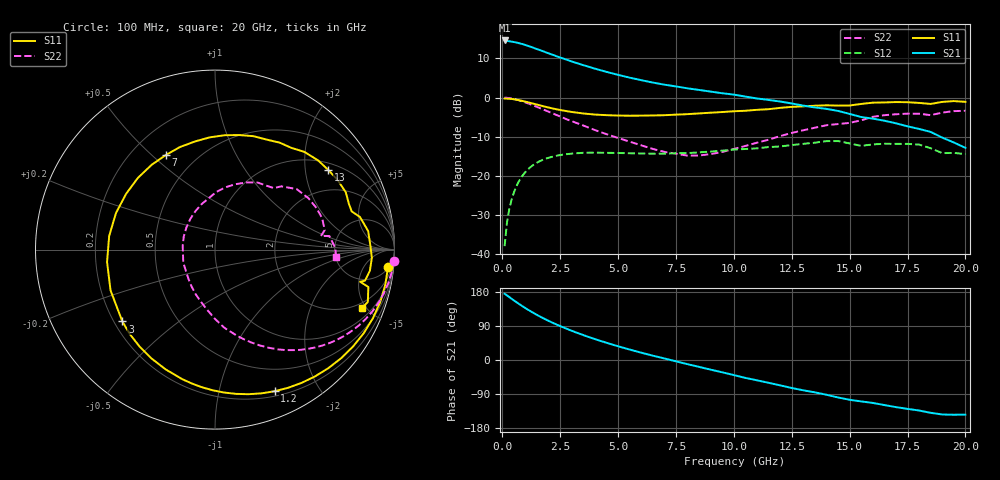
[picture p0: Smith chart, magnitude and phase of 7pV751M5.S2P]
! Infineon Technologies  Discrete & RF Semiconductors
! bfp620
! VCE = 0.75 V,  IC =  1.5 mA
! Common Emitter S-Parameters:  Sep 2002
# GHz  S  MA  R  50
!  f  S11  S21  S12  S22
! GHz  MAG  ANG  MAG  ANG  MAG  ANG  MAG  ANG
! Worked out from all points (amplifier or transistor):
!   59 points, 100 MHz to 20 GHz, reference 50 ohm
!   highest |S21| = 14.6 dB at 100 MHz (marker M1)
!   |S21| within 3 dB of that: start of sweep to 1.866 GHz
!   unconditionally stable (mu >= 1): 6.109 GHz to 15.89 GHz; 17.2 GHz to end of sweep
!   at 1 GHz: K = 0.14, MSG = 16.3 dB, |S12| = -19.1 dB
!   at 5.5 GHz: K = 0.90, MSG = 9.7 dB, |S12| = -14.3 dB
!   at 20 GHz: K = 1.78, MAG = -4.3 dB, |S12| = -14.5 dB
!   S11 on the Smith chart (normalised r, x): 100 MHz: 6, -18; 1.2 GHz: 0.25, -1.48; 3 GHz: 0.23, -0.33; 7 GHz: 0.34, +0.55; 13 GHz: 1.22, +2.67; 20 GHz: 1.62, -4.71
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0.1  0.9688 -5.6  5.381 174.8  0.0125 87.2  0.9982 -3.8
0.2  0.969 -11.7  5.315 170.6  0.0247 83.3  0.9921 -7.5
0.3  0.9657 -17.7  5.257 166.1  0.037 79.7  0.9831 -11.1
0.7  0.9274 -40.7  4.986 148.8  0.0829 65.3  0.9247 -24.7
0.9  0.9002 -51.6  4.802 140.7  0.1025 58.4  0.8862 -30.8
1.2  0.8562 -67.2  4.489 129.4  0.1274 49.0  0.8228 -39.3
1.6  0.7976 -86.5  4.071 115.6  0.1522 38.2  0.7372 -49.2
2.2  0.7221 -112.3  3.502 97.5  0.1759 25.0  0.6225 -61.4
2.6  0.6844 -127.9  3.179 86.9  0.1854 17.8  0.5551 -68.7
3  0.6532 -142.2  2.893 77.0  0.1914 11.2  0.4979 -75.4
3.5  0.6249 -158.6  2.599 65.7  0.1962 4.2  0.4385 -83.2
4  0.6053 -173.5  2.343 55.2  0.1968 -2.0  0.3834 -90.4
5  0.5881 159.8  1.952 36.2  0.195 -11.0  0.3037 -104.5
6  0.5867 137.1  1.67 19.3  0.1921 -17.8  0.2445 -122.1
7  0.5939 117.5  1.462 4.1  0.1911 -22.3  0.2015 -143.3
8.5  0.6259 92.8  1.251 -18.2  0.1986 -28.6  0.1812 172.9
10.5  0.6774 64.7  1.028 -47.3  0.2194 -39.6  0.2401 117.2
13  0.7717 35.1  0.788 -80.0  0.2553 -55.5  0.3811 72.8
13.5  0.7855 29.5  0.747 -85.4  0.2644 -60.0  0.4109 65.5
15  0.7907 15.6  0.617 -105.0  0.2585 -80.3  0.4734 46.4
17  0.8752 -3.0  0.468 -124.3  0.2553 -92.3  0.6109 22.3
20  0.8814 -21.6  0.227 -144.1  0.1888 -115.3  0.6765 -3.6
